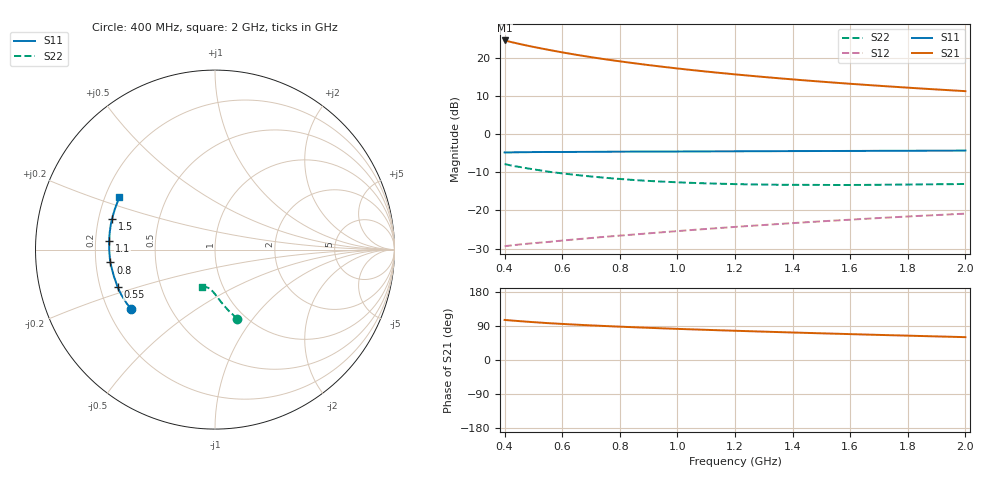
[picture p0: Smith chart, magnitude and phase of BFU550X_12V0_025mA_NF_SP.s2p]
! Filename:  P:\Prog\Test\Noise\ATS_data\Testdata_Net\BFU550X attenuator noise\BFU550X_APG2013_44_C05_12p0V_025mA_NF_CM01_D.sf
! Date/Time: Fri 26/Jul/2013 14:34:25
! BFU550X_APG2013_44_C05_12p0V_1to35mA_NF_CM01_Bias7_R.sf
! Noise Parameter Data File
! BFU550X_APG2013_44_C05_12p0V_1to35mA_NF_CM01
! Date/time: Mon Jul 22 11:28:10 2013
! VAR V_out= 12.001000
! VAR I_out= 25.000000
! VAR V_in= 0.757300
! VAR I_in= 0.243500
! Device data file deembeded for feedlines and parallel
! Original file: \BFU550X attenuator noise\BFU550X_APG2013_44_C05_12p0V_025mA_NF_CM01_R.sf
! Feed-files: PR005V01_100713_Feed1.s2p, PR005V01_100713_Feed2.s2p
! Parallel-file: PR005V01_100713_Par.s2p
# MHz S MA R 50
!  Freq-MHz  S11-mag  S11-arg  S21-mag  S21-arg  S12-mag  S12-arg  S22-mag  S22-arg
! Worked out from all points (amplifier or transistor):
!   37 points, 400 MHz to 2 GHz, reference 50 ohm
!   highest |S21| = 24.5 dB at 400 MHz (marker M1)
!   |S21| within 3 dB of that: start of sweep to 592 MHz
!   unconditionally stable (mu >= 1): 1.507 GHz to end of sweep
!   at 500 MHz: K = 0.64, MSG = 25.7 dB, |S12| = -28.6 dB
!   at 1.1 GHz: K = 0.93, MSG = 20.6 dB, |S12| = -24.8 dB
!   at 2 GHz: K = 1.04, MAG = 14.8 dB, |S12| = -20.8 dB
!   lowest NFmin = 1.19 dB at 440 MHz
!   S11 on the Smith chart (normalised r, x): 400 MHz: 0.30, -0.29; 550 MHz: 0.27, -0.17; 800 MHz: 0.26, -0.06; 1.1 GHz: 0.26, +0.04; 1.5 GHz: 0.26, +0.14; 2 GHz: 0.26, +0.24
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400  0.5744 -144.8  16.71 105.8  0.03408 47.2  0.4037 -72.2
420  0.5735 -146.9  16.02 104.5  0.03476 47.4  0.3892 -73.6
440  0.5762 -149.0  15.4 103.2  0.03545 47.4  0.3762 -74.5
460  0.5768 -150.9  14.82 102.1  0.03612 47.5  0.3667 -75.8
500  0.5796 -154.5  13.77 99.9  0.03732 47.7  0.3453 -77.8
550  0.5816 -158.8  12.66 97.3  0.03864 48.3  0.3216 -80.1
600  0.5809 -162.1  11.68 95.2  0.04036 48.9  0.3052 -82.0
650  0.5827 -165.2  10.84 93.2  0.04195 49.5  0.2903 -83.8
700  0.5834 -168.0  10.11 91.3  0.04358 50.1  0.2778 -85.4
750  0.5853 -170.6  9.474 89.6  0.04525 50.7  0.2672 -86.8
800  0.5872 -173.0  8.916 88.0  0.0468 51.2  0.2579 -88.4
850  0.588 -175.3  8.415 86.4  0.04843 51.8  0.2498 -89.7
900  0.588 -177.4  7.961 84.9  0.05015 52.5  0.2432 -90.9
950  0.5892 -179.4  7.56 83.5  0.05188 52.9  0.2378 -92.1
1000  0.5897 178.7  7.193 82.2  0.05364 53.4  0.2334 -93.2
1100  0.5914 175.3  6.554 79.6  0.05724 54.2  0.226 -95.2
1200  0.5934 172.1  6.021 77.2  0.06087 54.8  0.221 -97.1
1350  0.5963 167.5  5.362 73.7  0.06638 55.6  0.2166 -99.8
1500  0.5986 163.4  4.834 70.4  0.07199 55.9  0.2155 -102.2
1600  0.6 160.7  4.534 68.3  0.0757 56.1  0.2152 -103.7
1750  0.6021 157.0  4.148 65.2  0.08141 56.2  0.2174 -106.0
2000  0.6066 151.3  3.63 60.3  0.09079 56.0  0.2219 -109.5
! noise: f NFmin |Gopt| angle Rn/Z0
400  1.197  0.2785  -175.2  0.086
460  1.203  0.288  -176.2  0.0771
600  1.217  0.2873  -173.4  0.081
800  1.226  0.3079  -170.6  0.0783
1000  1.261  0.3183  -167.8  0.0776
1200  1.285  0.3273  -167.3  0.0784
1400  1.308  0.3503  -162.3  0.0793
1600  1.343  0.3545  -158.4  0.0873
1800  1.365  0.3531  -158.6  0.0872
2000  1.396  0.376  -154.7  0.0905
